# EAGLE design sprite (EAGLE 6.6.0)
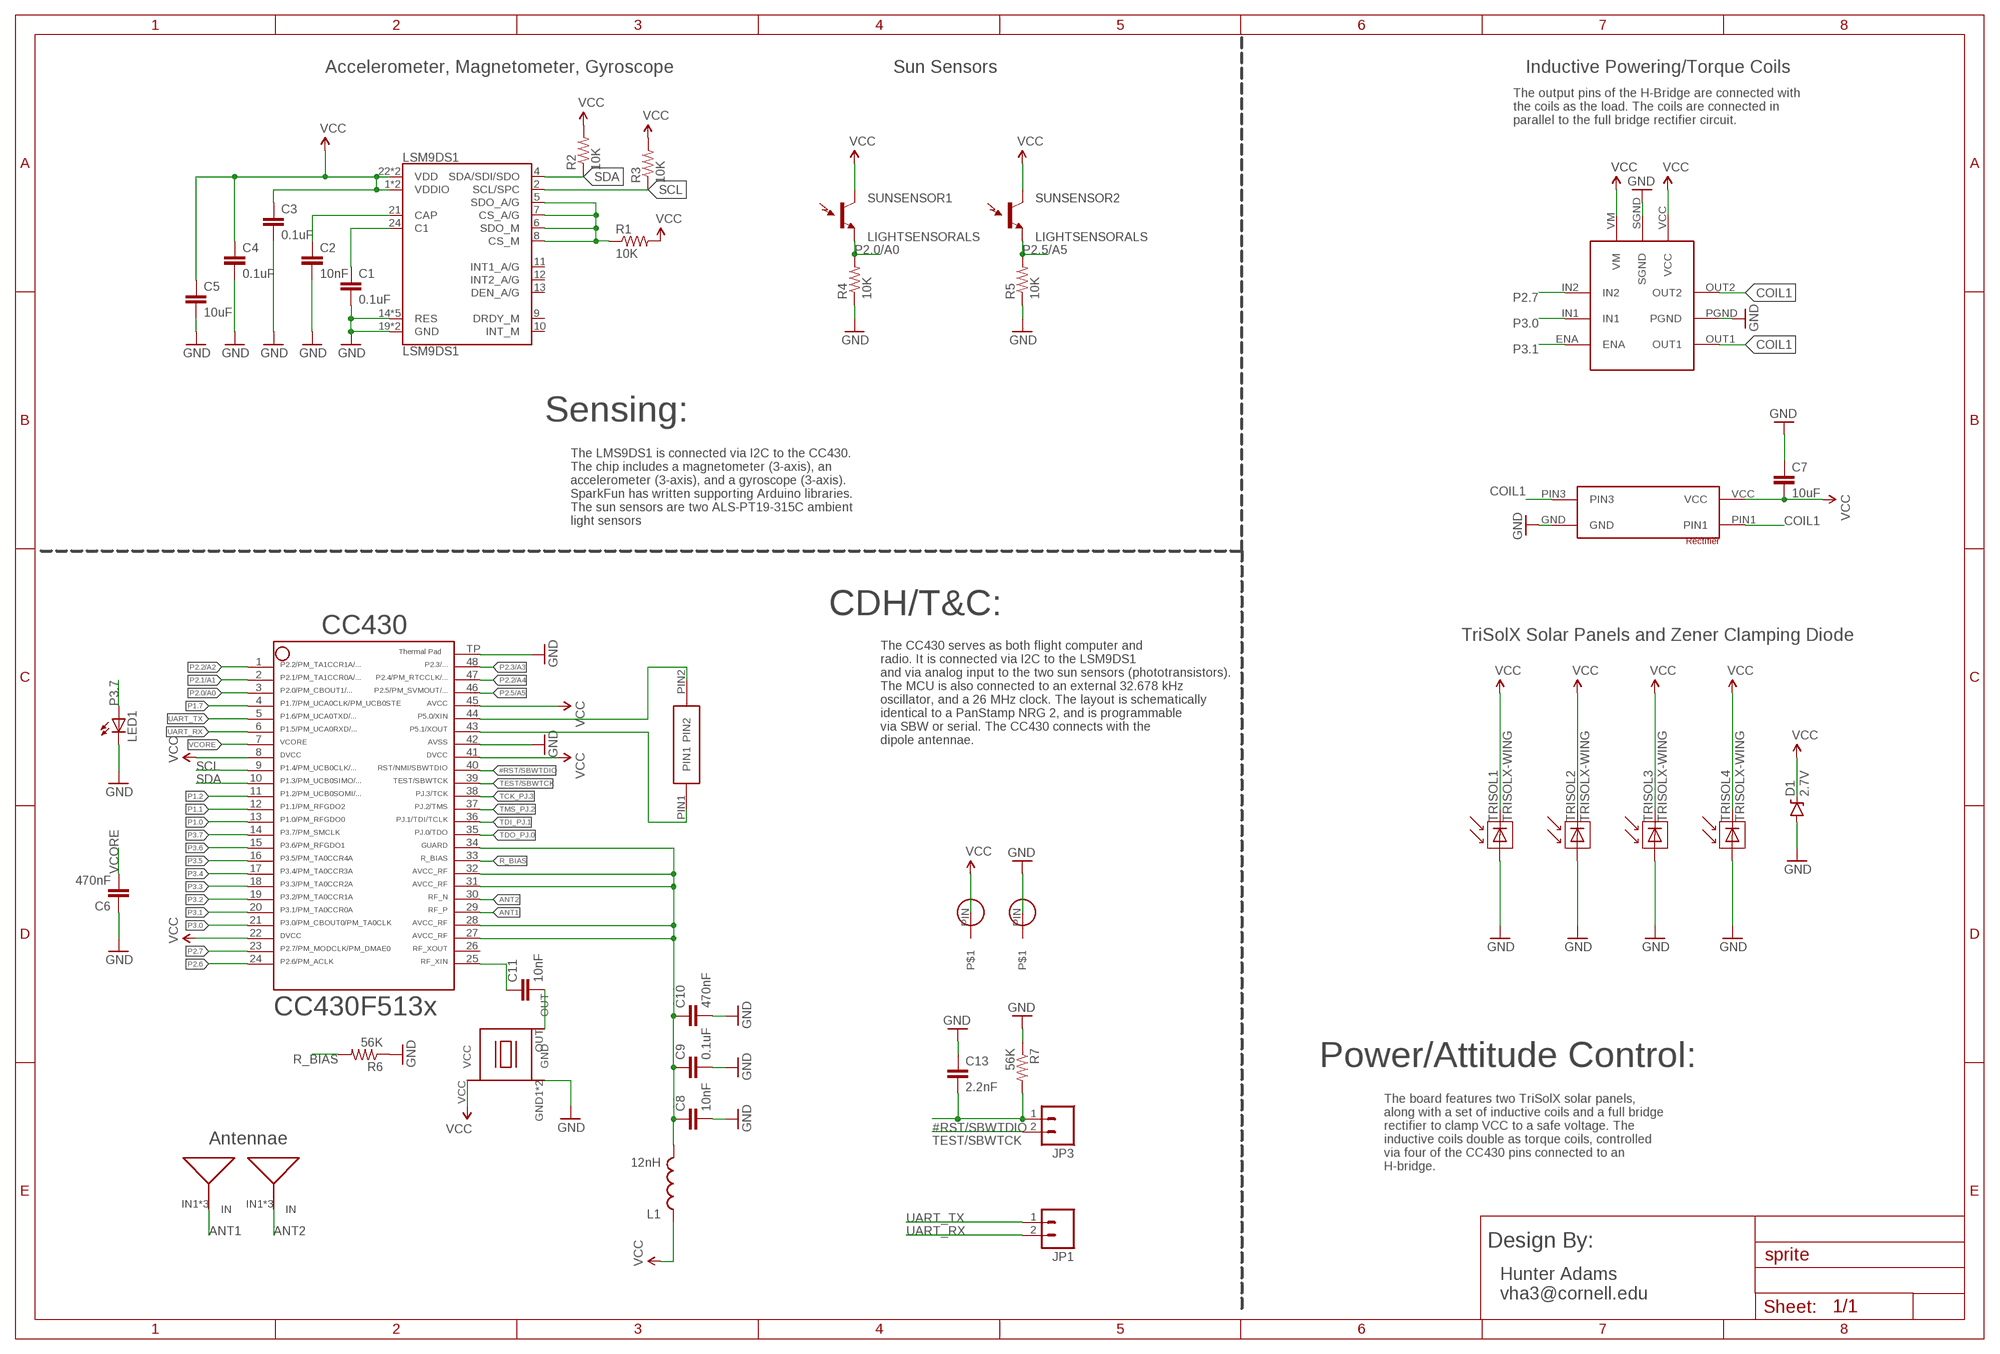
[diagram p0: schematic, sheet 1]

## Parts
32KHZ  SPRITECRYSTALSPRITECRYSTAL  [SPRITECRYSTAL]
ANTENNA1  ANTENNA  [ANTENNA]
ANTENNA2  ANTENNA  [ANTENNA]
C1  0.1uF  CAP0805  [0805]
C2  10nF  CAP0805  [0805]
C3  0.1uF  CAP0805  [0805]
C4  0.1uF  CAP0805  [0805]
C5  10uF  CAP0805  [0805]
C6  470nF  CAP0805  [0805]
C7  10uF  CAP0805  [0805]
C8  10nF  CAP0805  [0805]
C9  0.1uF  CAP0805  [0805]
C10  470nF  CAP0805  [0805]
C11  10nF  CAP0805  [0805]
C13  2.2nF  CAP0805  [0805]
CC430  CC430F513X---RGZ48  [RGZ48]
D1  2.7V  DIODE-ZENER3.3V  [SOD-323]
GNDPIN  SPRITE_PIN  [SPRITE_PIN]
H-BRIDGE  LV8417CS  [LV8417CS]
JP1  M02PTH  [1X02]
JP3  M02PTH  [1X02]
L1  12nH  INDUCTOR0402  [C0402]
LED1  LED0603  [LED-0603]
LSM9DS1  LSM9DS1  [LGA24-8X4]
R1  10K  RESISTOR0805-RES  [0805]
R2  10K  RESISTOR0805-RES  [0805]
R3  10K  RESISTOR0805-RES  [0805]
R4  10K  RESISTOR0805-RES  [0805]
R5  10K  RESISTOR0805-RES  [0805]
R6  56K  RESISTOR0805-RES  [0805]
R7  56K  RESISTOR0805-RES  [0805]
RECTIFIER  NSR1030QMUTAG  [NSR1030QMUTAG]
SUNSENSOR1  LIGHTSENSORALS  [ALS-PT19]
SUNSENSOR2  LIGHTSENSORALS  [ALS-PT19]
TRISOL1  TRISOLX-WING  [TRISOLX-T01]
TRISOL2  TRISOLX-WING  [TRISOLX-T01]
TRISOL3  TRISOLX-WING  [TRISOLX-T01]
TRISOL4  TRISOLX-WING  [TRISOLX-T01]
TXCO  TCXO_7Z  [TXC_7Z]
VCCPIN  SPRITE_PIN  [SPRITE_PIN]

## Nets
#RST/SBWTDIO: C13.2 CC430.40 JP3.1 R7.2
ANT1: ANTENNA1.IN1(IN) ANTENNA1.IN2(IN) ANTENNA1.IN3(IN) CC430.29
ANT2: ANTENNA2.IN1(IN) ANTENNA2.IN2(IN) ANTENNA2.IN3(IN) CC430.30
COIL1: H-BRIDGE.OUT1 H-BRIDGE.OUT2 RECTIFIER.PIN1 RECTIFIER.PIN3
GND: C1.2 C2.2 C3.2 C4.2 C5.2 C6.1 C7.1 C8.2 C9.2 C10.2 C13.1 CC430.42 CC430.TP D1.A GNDPIN.PIN H-BRIDGE.PGND H-BRIDGE.SGND LED1.C LSM9DS1.14(RES) LSM9DS1.15(RES) LSM9DS1.16(RES) LSM9DS1.17(RES) LSM9DS1.18(RES) LSM9DS1.19(GND) LSM9DS1.20(GND) R4.1 R5.1 R6.1 R7.1 RECTIFIER.GND TRISOL1.P$3(A) TRISOL2.P$3(A) TRISOL3.P$3(A) TRISOL4.P$3(A) TXCO.GND1(GND) TXCO.GND2(GND)
GUARD: C8.1 C9.1 C10.1 CC430.27 CC430.28 CC430.31 CC430.32 CC430.34 L1.2
N$1: C1.1 LSM9DS1.24(C1)
N$2: C2.1 LSM9DS1.21(CAP)
N$3: LSM9DS1.5(SDO_A/G) LSM9DS1.6(SDO_M) LSM9DS1.7(CS_A/G) LSM9DS1.8(CS_M) R1.1
N$4: C11.1 CC430.25
N$5: C11.2 TXCO.OUT
N$7: 32KHZ.PIN2 CC430.44
N$8: 32KHZ.PIN1 CC430.43
P1.0: CC430.13
P1.1: CC430.12
P1.2: CC430.11
P1.7: CC430.4
P2.0/A0: CC430.3 R4.2 SUNSENSOR1.E(E1)
P2.1/A1: CC430.2
P2.2/A2: CC430.1
P2.2/A4: CC430.47
P2.3/A3: CC430.48
P2.5/A5: CC430.46 R5.2 SUNSENSOR2.E(E1)
P2.6: CC430.24
P2.7: CC430.23 H-BRIDGE.IN2
P3.0: CC430.21 H-BRIDGE.IN1
P3.1: CC430.20 H-BRIDGE.ENA
P3.2: CC430.19
P3.3: CC430.18
P3.4: CC430.17
P3.5: CC430.16
P3.6: CC430.15
P3.7: CC430.14 LED1.A
R_BIAS: CC430.33 R6.2
SCL: CC430.9 LSM9DS1.2(SCL/SPC) R3.1
SDA: CC430.10 LSM9DS1.4(SDA/SDI/SDO) R2.1
TCK_PJ.3: CC430.38
TDI_PJ.1: CC430.36
TDO_PJ.0: CC430.35
TEST/SBWTCK: CC430.39 JP3.2
TMS_PJ.2: CC430.37
UART_RX: CC430.6 JP1.2
UART_TX: CC430.5 JP1.1
VCC: C3.1 C4.1 C5.1 C7.2 CC430.8 CC430.22 CC430.41 CC430.45 D1.C H-BRIDGE.VCC H-BRIDGE.VM L1.1 LSM9DS1.1(VDDIO) LSM9DS1.3(VDDIO) LSM9DS1.22(VDD) LSM9DS1.23(VDD) R1.2 R2.2 R3.2 RECTIFIER.VCC SUNSENSOR1.C(C1) SUNSENSOR2.C(C1) TRISOL1.P$2(C) TRISOL2.P$2(C) TRISOL3.P$2(C) TRISOL4.P$2(C) TXCO.VCC VCCPIN.PIN
VCORE: C6.2 CC430.7
Unconnected: CC430.26 LSM9DS1.9(DRDY_M) LSM9DS1.10(INT_M) LSM9DS1.11(INT1_A/G) LSM9DS1.12(INT2_A/G) LSM9DS1.13(DEN_A/G)

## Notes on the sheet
- Accelerometer, Magnetometer, Gyroscope | Sun Sensors | Inductive Powering/Torque Coils
- The output pins of the H-Bridge are connected with
  the coils as the load. The coils are connected in 
  parallel to the full bridge rectifier circuit.
- Sensing:
- The LMS9DS1 is connected via I2C to the CC430. 
  The chip includes a magnetometer (3-axis), an 
  accelerometer (3-axis), and a gyroscope (3-axis). 
  SparkFun has written supporting Arduino libraries. 
  The sun sensors are two ALS-PT19-315C ambient 
  light sensors
- CDH/T&C:
- TriSolX Solar Panels and Zener Clamping Diode
- The CC430 serves as both flight computer and
  radio. It is connected via I2C to the LSM9DS1 
  and via analog input to the two sun sensors (phototransistors). 
  The MCU is also connected to an external 32.678 kHz 
  oscillator, and a 26 MHz clock. The layout is schematically 
  identical to a PanStamp NRG 2, and is programmable 
  via SBW or serial. The CC430 connects with the 
  dipole antennae.
- Power/Attitude Control:
- Antennae
- The board features two TriSolX solar panels, 
  along with a set of inductive coils and a full bridge 
  rectifier to clamp VCC to a safe voltage. The 
  inductive coils double as torque coils, controlled 
  via four of the CC430 pins connected to an 
  H-bridge.
- Design By:
- Hunter Adams
  vha3@cornell.edu

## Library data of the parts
32KHZ = SpriteCrystal:SPRITECRYSTAL
ANTENNA1 ANTENNA2 = SpriteAntenna:ANTENNA
C1-C11 C13 = SparkFun:CAP: Capacitor
CC430 = TI_MSP430_v16:CC430F513X---RGZ48: ***CC430F513X***RGZ48 ** ** Rev 1.0 ** 06/2010 * http://focus.ti.com/docs/prod/folders/print/cc430f5137.html
D1 = SparkFun-DiscreteSemi:DIODE-ZENER: Zener Diode; PROD_ID: DIO-11284; VALUE: 3.3V
GNDPIN VCCPIN = SpritePin:SPRITE_PIN
H-BRIDGE = lv8417cs:LV8417CS
JP1 JP3 = SparkFun:M02: Header 2
L1 = SparkFun:INDUCTOR: Inductors
LED1 = SparkFun:LED: LEDs
LSM9DS1 = SparkFun-Sensors:LSM9DS1: LSM9DS1 3D accelerometer, gyroscope & magnetometer The LSM9DS1 is a system-in-package featuring a 3D digital linear acceleration sensor, a 3D digital angular rate sensor, and a 3D digital magnetic sensor. The LSM9DS1 has a linear acceleration full scale of ±2g/±4g/±8/±16 g, a magnetic field full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; PROD_ID: IC-12536
R1-R7 = SparkFun:RESISTOR: Resistor
RECTIFIER = NSR1030QMUTAG:NSR1030QMUTAG
SUNSENSOR1 SUNSENSOR2 = SparkFun-Sensors:LIGHTSENSOR: Ambient Light Sensor; PROD_ID: IC-11836
TRISOL1-TRISOL4 = TriSolX_QzQube:TRISOLX-WING
TXCO = SpriteTCXO:TCXO_7Z

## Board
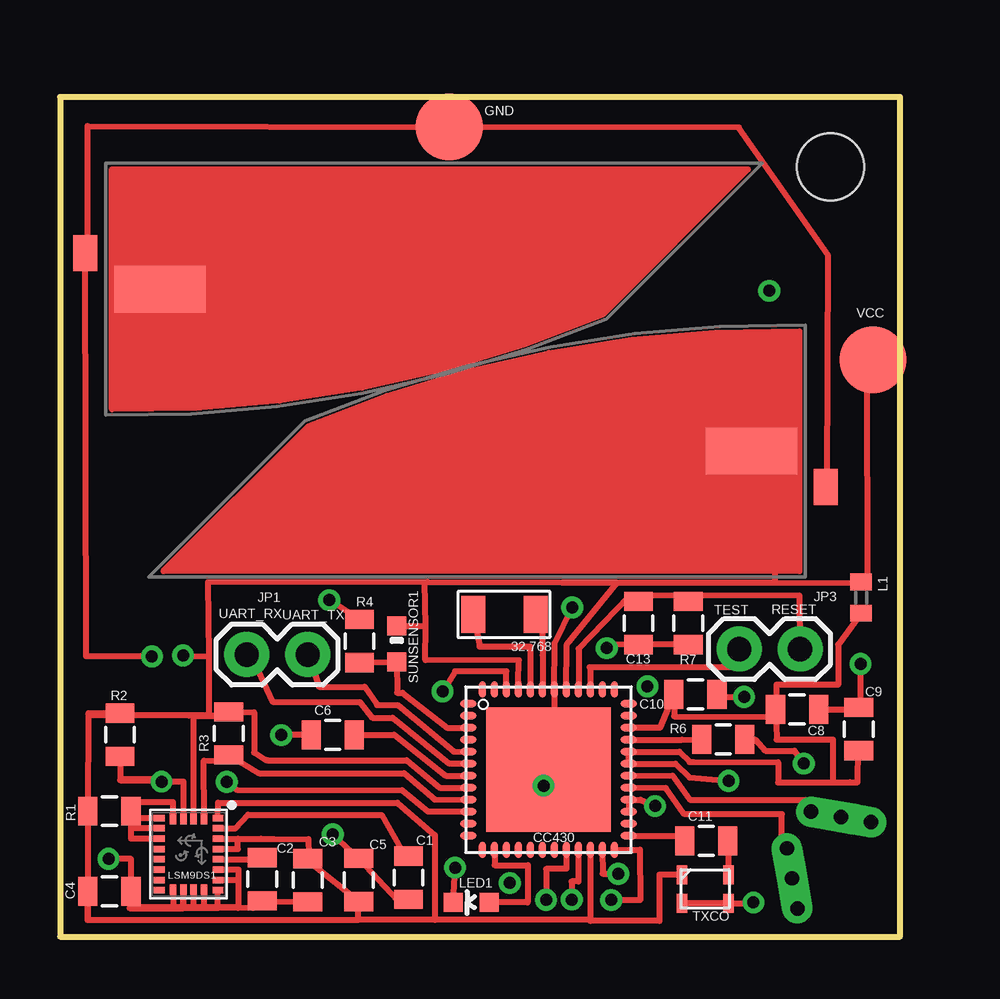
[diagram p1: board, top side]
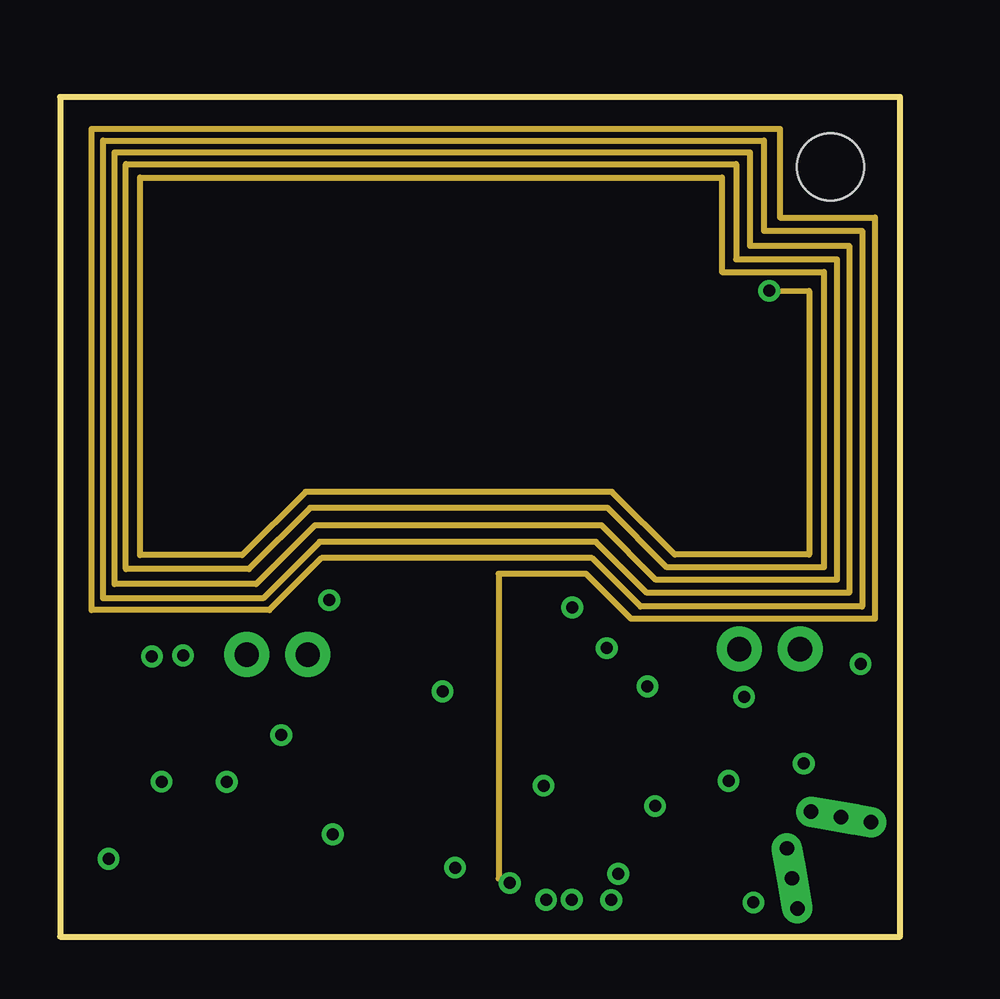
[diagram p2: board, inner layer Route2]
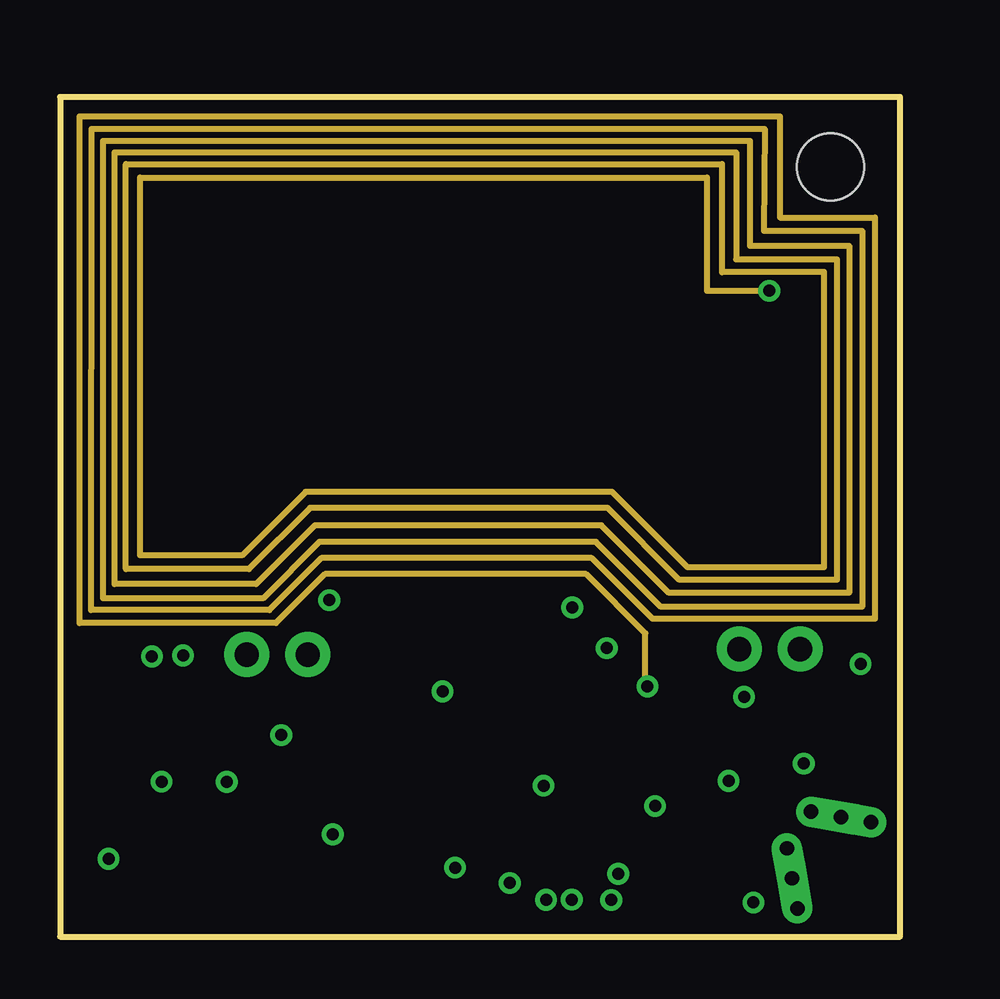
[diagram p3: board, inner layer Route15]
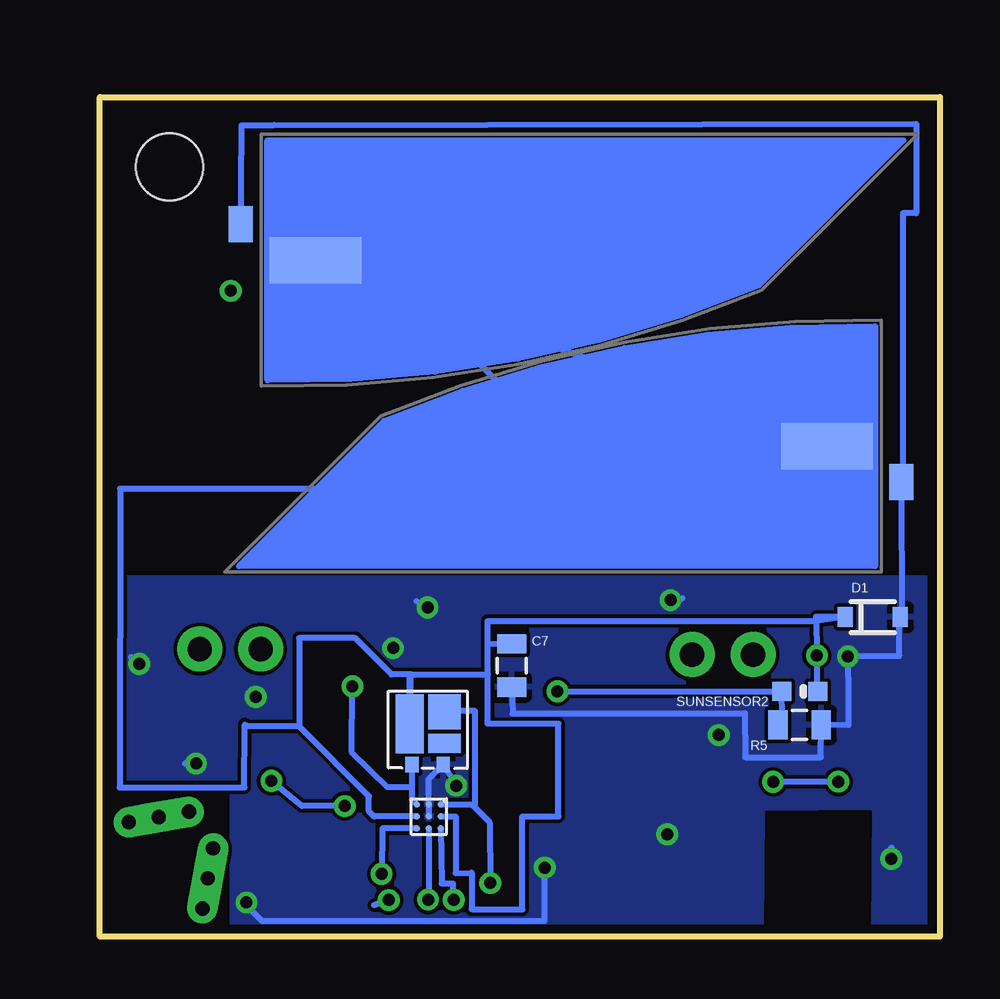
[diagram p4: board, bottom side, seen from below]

Size 35 x 35 mm. Coordinates in mm from the lower left corner, seen from the top.
Outline: 0,0 35,0 35,35 0,35 0,0
Copper layers (1*2*15*16): Top 0.035559375mm / dielectric 1.501140625mm / Route2 0.035559375mm / dielectric 0.149859375mm / Route15 0.035559375mm / dielectric 0.200659375mm / Bottom 0.035559375mm
Design rules "typical_4pcb *": minimum track width 10mil, minimum drill 15mil, track to track 6mil, track to pad 6mil, pad to pad 6mil, via to via 6mil, smd to smd 6mil, copper to edge 15mil, drill to drill 8mil, minimum pad ring 10mil, minimum via ring 8mil, stop-mask expansion 4mil, vias tented up to drill 0mil, thermal gap 10mil
Holes 2.8 mm at 32.1,32.1

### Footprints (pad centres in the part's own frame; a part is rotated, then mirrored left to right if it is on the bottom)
SPRITECRYSTAL = smd 1 x 1.55: PIN1 -1.3,0; PIN2 1.3,0
ANTENNA = drill 0.6 pad 1.27 square: IN1 0,0 | drill 0.6 pad 1.27 offset: IN2 1.27,0; IN3 -1.27,0
0805 = smd 0.8 x 1.2: 1 -0.9,0; 2 0.9,0
RGZ48 = smd 0.7 x 0.3: 1 -3.35,2.75; 2 -3.35,2.25; 3 -3.35,1.75; 4 -3.35,1.25; 5 -3.35,0.75; 6 -3.35,0.25; 7 -3.35,-0.25; 8 -3.35,-0.75; 9 -3.35,-1.25; 10 -3.35,-1.75; 11 -3.35,-2.25; 12 -3.35,-2.75; 25 3.35,-2.75; 26 3.35,-2.25; 27 3.35,-1.75; 28 3.35,-1.25; 29 3.35,-0.75; 30 3.35,-0.25; 31 3.35,0.25; 32 3.35,0.75; 33 3.35,1.25; 34 3.35,1.75; 35 3.35,2.25; 36 3.35,2.75 | smd 0.3 x 0.7: 13 -2.75,-3.35; 14 -2.25,-3.35; 15 -1.75,-3.35; 16 -1.25,-3.35; 17 -0.75,-3.35; 18 -0.25,-3.35; 19 0.25,-3.35; 20 0.75,-3.35; 21 1.25,-3.35; 22 1.75,-3.35; 23 2.25,-3.35; 24 2.75,-3.35; 37 2.75,3.35; 38 2.25,3.35; 39 1.75,3.35; 40 1.25,3.35; 41 0.75,3.35; 42 0.25,3.35; 43 -0.25,3.35; 44 -0.75,3.35; 45 -1.25,3.35; 46 -1.75,3.35; 47 -2.25,3.35; 48 -2.75,3.35 | smd 5.2 x 5.2: TP 0,0
SOD-323 = smd 0.63 x 0.83: A 1.15,0; C -1.15,0
SPRITE_PIN = smd 2.794 x 2.794: PIN 0,0
LV8417CS = smd 0.27 x 0.27: ENA 0.5,-0.5; IN1 0,-0.5; IN2 -0.5,-0.5; OUT1 0.5,0.5; OUT2 -0.5,0.5; PGND 0,0.5; SGND 0,0; VCC 0.5,0; VM -0.5,0
1X02 = drill 1.016 pad 1.88: 1 0,0; 2 2.54,0
C0402 = smd 0.7 x 0.9: 1 -0.65,0; 2 0.65,0
LED-0603 = smd 0.8 x 0.8: A 0,-0.75; C 0,0.75
LGA24-8X4 = smd 0.27 x 0.45: 1 -1.505,1.225; 6 -1.505,-1.225; 7 -1.075,-1.225; 8 -0.645,-1.225; 9 -0.215,-1.225; 10 0.215,-1.225; 11 0.645,-1.225; 12 1.075,-1.225; 13 1.505,-1.225; 18 1.505,1.225; 19 1.075,1.225; 20 0.645,1.225; 21 0.215,1.225; 22 -0.215,1.225; 23 -0.645,1.225; 24 -1.075,1.225 | smd 0.45 x 0.27: 2 -1.475,0.645; 3 -1.475,0.215; 4 -1.475,-0.215; 5 -1.475,-0.645; 14 1.475,-0.645; 15 1.475,-0.215; 16 1.475,0.215; 17 1.475,0.645
NSR1030QMUTAG = smd 0.55 x 0.633: GND -0.65,1.335; PIN3 0.65,1.335 | smd 1.35 x 0.8: P$2 -0.706,0.453 | smd 1.35 x 1.45: PIN1 -0.7,-0.865 | smd 1.15 x 2.45: VCC 0.738,-0.365
ALS-PT19 = smd 0.8 x 0.8: C -0.75,0; E 0.75,0
TRISOLX-T01 = smd 3.81 x 1.93: P$2 -2,5 | smd 1 x 1.5: P$3 1.1,3.5
TXC_7Z = smd 0.44 x 0.79: GND1 -0.97,-0.595; GND2 0.97,-0.595; OUT 0.97,0.595; VCC -0.97,0.595

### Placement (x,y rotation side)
32KHZ  18.52,13.44 180 top
ANTENNA1  30.51,2.44 100 top
ANTENNA2  32.55,5 170 top
C1  14.52,2.47 270 top
C2  8.43,2.4 270 top
C3  10.32,2.36 270 top
C4  2.06,1.9 0 top
C5  12.45,2.37 90 top
C6  11.36,8.41 0 top
C7  17.84,11.31 90 bottom
C8  30.71,9.48 0 top
C9  33.28,8.66 90 top
C10  26.48,10.11 0 top
C11  26.93,4 0 top
C13  24.11,13.08 90 top
CC430  20.35,6.97 0 top
D1  2.8,13.33 0 bottom
GNDPIN  16.22,33.76 0 top
H-BRIDGE  21.29,5.02 0 bottom
JP1  10.32,11.77 180 top
JP3  30.84,11.99 180 top
L1  33.38,14.14 270 top
LED1  17.13,1.44 90 top
LSM9DS1  5.36,3.45 270 top
R1  2.06,5.24 180 top
R2  2.5,8.42 90 top
R3  7.03,8.48 90 top
R4  12.48,12.32 270 top
R5  5.85,8.83 180 bottom
R6  27.63,8.22 180 top
R7  26.18,13.08 90 top
RECTIFIER  21.35,8.51 180 bottom
SUNSENSOR1  14.04,12.2 270 top
SUNSENSOR2  5.84,10.23 180 bottom
TRISOL1  2.16,31.99 180 top
TRISOL2  30.81,15.24 0 top
TRISOL3  2.7,15.45 0 bottom
TRISOL4  28.03,33.2 180 bottom
TXCO  26.88,2 0 top
VCCPIN  33.87,24.05 0 top

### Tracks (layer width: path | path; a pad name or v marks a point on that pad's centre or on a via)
#RST/SBWTDIO
  Top 0.254: R7.2 25.97,13.98 25.97,14.21 24.61,14.22 C13.2 23.7,14.18 | 23.7,14.18 21.61,12.01 21.61,10.32 CC430.40 | JP3.1 30.82,14.22 24.43,14.21 24.28,14.06 23.7,14.18
ANT1
  Top 0.254: ANTENNA1.IN3 ANTENNA1.IN1 ANTENNA1.IN2 30.08,3.64 30.08,5.11 26.02,5.11 25.24,6.2 23.72,6.2 CC430.29
ANT2
  Top 0.254: ANTENNA2.IN3 ANTENNA2.IN1 ANTENNA2.IN2 31.29,5.7 26.25,5.71 25.52,6.73 CC430.30
COIL1  (via drill 0.5)
  Route2 0.254: v18.74,2.24 18.28,2.43 18.28,15.13 21.92,15.13 23.79,13.26 33.95,13.26 33.95,29.99 30,29.99 30,33.68 1.32,33.68 1.32,13.62 8.72,13.62 10.89,15.79 22.17,15.79 24.2,13.76 33.42,13.76 33.42,29.43 29.33,29.43 29.33,33.19 1.8,33.19 1.8,14.11 8.46,14.11 10.81,16.46 22.33,16.46 24.46,14.34 32.88,14.34 32.88,28.81 28.74,28.81 28.74,32.7 2.27,32.7 2.27,14.7 8.17,14.7 10.62,17.15 22.56,17.15 24.83,14.88 32.37,14.88 32.37,28.24 28.17,28.24 28.17,32.21 2.75,32.21 2.75,15.33 7.87,15.33 10.42,17.88 22.82,17.88 25.29,15.4 31.83,15.4 31.83,27.71 27.57,27.71 27.57,31.65 3.34,31.65 3.34,15.91 7.59,15.91 10.23,18.55 23,18.55 25.62,15.93 | v29.55,26.93 31.21,26.92 31.21,15.93 25.62,15.93 | 25.62,15.93
  Route15 0.254: v24.48,10.44 24.39,10.51 | 24.39,10.51 24.23,10.63 | 24.39,10.51 24.39,12.65 21.92,15.12 | 21.92,15.12 | 21.92,15.12 11.04,15.12 9,13.08 0.82,13.08 0.82,34.21 29.99,34.21 29.99,29.99 33.96,29.99 33.96,13.26 24.69,13.26 22.17,15.78 10.88,15.78 8.72,13.62 1.29,13.62 1.32,33.68 29.36,33.68 29.33,29.43 33.42,29.43 33.42,13.76 25.03,13.76 22.33,16.46 10.81,16.46 8.46,14.11 1.8,14.11 1.8,33.19 28.74,33.19 28.74,28.8 32.88,28.8 32.88,14.34 25.37,14.34 22.56,17.15 10.62,17.15 8.17,14.7 2.27,14.7 2.27,32.7 28.17,32.7 28.17,28.24 32.37,28.24 32.37,14.88 25.81,14.88 22.82,17.88 10.42,17.88 7.87,15.33 2.75,15.33 2.75,32.21 27.58,32.21 27.58,27.72 | 27.58,27.72 27.58,27.69 | 27.58,27.72 31.83,27.72 31.83,15.4 26.15,15.4 23.01,18.55 10.23,18.55 7.59,15.9 3.34,15.9 3.34,31.65 26.95,31.65 26.95,26.93 v29.55,26.93
  Bottom 0.254: H-BRIDGE.OUT1 19.5,5.51 | 19.5,5.51 19.36,5.51 19.36,9.41 20.65,9.41 RECTIFIER.PIN1 | 19.5,5.51 18.77,4.77 v18.74,2.24 | 22,6.24 22,5.72 H-BRIDGE.OUT2 | 22,6.24 23.02,6.24 24.5,7.68 v24.48,10.44 | RECTIFIER.PIN3 22,6.24
GND  (via drill 0.5)
  Top 0.254: 6.55,1.97 LSM9DS1.18 6.58,1.2 | 7.42,1.19 8.05,1.2 8.06,1.5 C2.2 8.21,1.48 C3.2 | 7.42,1.19 6.58,1.2 | C1.2 14.08,1.52 C5.2 v11.36,4.27 | C4.2 2.9,1.2 4.69,1.2 | 4.69,1.2 5.14,1.2 LSM9DS1.15 5.13,1.2 5.56,1.2 | C9.2 33.65,9.48 C8.2 33.36,9.48 v33.36,11.37 | R7.1 C13.1 22.89,12.18 v22.79,12.04 | 7.43,2.37 7.43,2.8 LSM9DS1.20 7.42,2.8 7.42,1.22 2.96,1.22 2.96,3.25 v2.02,3.25 | 7.43,2.37 7.42,1.19 | LSM9DS1.19 7.43,2.37 | LSM9DS1.14 4.71,1.22 4.69,1.2 | 5.56,1.2 5.99,1.2 | 5.99,1.2 6.58,1.2 | LSM9DS1.16 5.56,1.2 | LSM9DS1.17 5.99,1.2 | TRISOL2.P$3 31.97,18.94 32.01,28.42 28.29,33.73 16.32,33.74 GNDPIN.PIN 1.15,33.8 1.15,28.65 TRISOL1.P$3 1.09,11.69 v3.83,11.69 | v21.35,13.73 20.61,12.23 CC430.42 20.6,9.3 20.59,9.3 CC430.TP 20.35,6.43 20.09,6.17 v20.15,6.3 | LED1.C v16.46,2.88 | C6.1 v9.21,8.41 | R4.1 v11.22,14.04 | C10.2 27.55,10.01 v28.5,10 | R6.1 28.96,8.22 29.39,7.75 30.6,7.75 v30.99,7.22 | 28.93,1.45 v28.89,1.43 28.96,1.4 TXCO.GND2 TXCO.GND1
  Bottom 0.254: C7.1 17.81,9.31 8.13,9.32 8.12,7.49 4.96,7.48 R5.1 3.82,8.81 3.82,10 v3.83,11.69 1.7,11.69 1.71,11.79 1.71,13.41 1.79,13.42 D1.A 1.59,13.24 TRISOL3.P$3 1.36,18.9 1.54,18.67 1.54,30.16 0.99,30.16 0.99,33.89 27.75,33.83 29.1,33.83 29.11,31.3 29.12,29.47 29.22,29.61 TRISOL4.P$3 | H-BRIDGE.SGND H-BRIDGE.PGND 21.29,6.59 RECTIFIER.GND v20.15,6.3 | 16.41,2.92 v16.46,2.88 16.47,0.66 16.62,0.66 28.25,0.66 29.04,1.44 v28.89,1.43 | v11.36,4.27 11.27,4.42 | v9.21,8.41 8.99,8.64 | v11.22,14.04 10.73,14.11 | v2.02,3.25 2.02,3.72 | v21.35,13.73 21.8,13.98 | v22.79,12.04 22.81,11.89 | v28.5,10 28.44,9.85 | v30.99,7.22 31.46,7.22 | v33.36,11.37 33.71,11.66
  pour Bottom: 0.21,14.95 34.8,14.95 34.8,6.09 29.49,6.09 29.49,0.25 7.44,0.21 7.41,5.38 2.72,5.42 2.76,0.12 -0.17,0.14 -0.17,14.97
GUARD  (via drill 0.5)
  Top 0.254: CC430.27 CC430.28 24.2,5.72 v24.8,5.45 | CC430.34 24.99,8.72 C10.1 25.59,9.19 29.86,9.17 | 29.86,9.17 29.86,9.08 C8.1 29.86,8.22 32.2,8.22 32.2,6.45 32.92,6.44 | L1.2 32.42,12.17 32.42,10.51 29.85,10.51 29.84,9.24 29.89,9.03 29.86,9.17 | 32.92,6.44 33.23,6.44 33.24,6.95 C9.1 | 32.92,6.44 29.92,6.44 29.92,7.28 26.4,7.29 26.24,7.29 25.81,7.72 CC430.32 CC430.31 25.64,7.22 26.22,6.64 v27.86,6.5
  Bottom 0.254: 27.78,6.66 v27.86,6.5 26.59,5.45 v24.8,5.45
N$1
  Top 0.254: LSM9DS1.24 6.56,4.53 7.3,4.52 7.83,5.09 13.4,5.08 14.22,3.65 14.36,3.37 C1.1
N$2
  Top 0.254: LSM9DS1.21 8,3.22 C2.1
N$3
  Top 0.254: 4.1,4.92 LSM9DS1.6 2.9,4.95 R1.1 | LSM9DS1.8 2.96,4.09 2.96,4.52 | 2.96,4.52 R1.1 | LSM9DS1.7 2.96,4.52 | LSM9DS1.5 4.71,5.61 3.33,5.61 arc90 R1.1
N$4
  Top 0.254: CC430.25 26.03,4.22 C11.1
N$5
  Top 0.254: C11.2 27.85,4 TXCO.OUT
N$7
  Top 0.254: 32KHZ.PIN2 17.49,12.09 19.6,12.09 CC430.44 | CC430.44
N$8
  Top 0.254: 32KHZ.PIN1 19.95,13.28 19.93,13.23 20.07,13.37 20.11,11.73 CC430.43
P2.0/A0
  Top 0.254: CC430.3 16.13,8.71 14.27,10.17 14.04,10.17 SUNSENSOR1.E 13.97,11.43 R4.2
P2.5/A5  (via drill 0.5)
  Top 0.254: CC430.46 18.6,11.06 16.46,11.06 v15.94,10.23
  Bottom 0.254: R5.2 6.58,9.19 SUNSENSOR2.E 6.55,10.23 v15.94,10.23
P2.6  (via drill 0.5)
  Top 0.254: CC430.24 24.17,3.63 24.18,1.53 23.31,1.52 v22.97,1.53
  Bottom 0.254: v22.97,1.53 23.57,1.32
P2.7  (via drill 0.5)
  Top 0.254: CC430.23 22.61,2.63 v23.26,2.63
  Bottom 0.254: 23.4,2.47 v23.26,2.63 23.23,4.51 H-BRIDGE.IN2
P3.0  (via drill 0.5)
  Top 0.254: CC430.21 21.6,2.31 21.32,2.3 v21.33,1.55
  Bottom 0.254: 21.43,1.55 v21.33,1.55 21.29,1.75 H-BRIDGE.IN1
P3.1  (via drill 0.5)
  Top 0.254: CC430.20 21.1,2.84 20.25,2.83 v20.25,1.54
  Bottom 0.254: H-BRIDGE.ENA 20.76,2.22 20.29,2.22 20.29,1.52 20.16,1.54 v20.25,1.54
P3.7
  Top 0.254: CC430.14 18.11,3.62 18.11,2.98 19.49,2.98 19.49,1.45 19.48,1.44 LED1.A
R_BIAS
  Top 0.254: CC430.33 25.91,8.22 R6.2
SCL
  Top 0.254: LSM9DS1.2 6,7.35 6.87,7.33 7.27,7.45 R3.1 8.3,6.82 14.34,6.82 15.61,5.72 CC430.9
SDA  (via drill 0.5)
  Top 0.254: LSM9DS1.4 5.14,6.48 v4.23,6.47 4.18,6.53 2.51,6.53 R2.1 2.51,6.58 4.19,6.58 v4.23,6.47 | v6.95,6.46 7.36,6.13 14.25,6.11 15.32,5.23 CC430.10
  Bottom 0.254: v4.23,6.47 v6.95,6.46
TEST/SBWTCK
  Top 0.254: JP3.2 28.28,11.23 22.07,11.23 22.1,11.18 CC430.39
UART_RX
  Top 0.254: JP1.2 7.89,11.91 8.86,9.79 12.5,9.79 13.02,9.13 13.86,9.13 16.19,7.23 CC430.6
UART_TX
  Top 0.254: JP1.1 10.8,10.42 12.68,10.42 12.69,10.41 13.21,9.66 14.07,9.66 16.4,7.72 16.99,7.71 CC430.5
VCC  (via drill 0.5)
  Top 0.254: 15.3,14.8 20.91,14.76 | 20.91,14.76 29.79,14.76 | 29.79,14.76 33.66,14.76 | 33.66,14.76 33.63,23.63 VCCPIN.PIN | 33.66,14.76 33.3,14.84 L1.1 | CC430.8 16.98,6.2 15.82,6.21 14.44,7.36 8.64,7.36 8.57,7.38 8.09,7.68 8.09,9.36 R3.2 7.24,9.3 7.25,9.21 5.57,9.23 LSM9DS1.3 5.58,9.22 7.12,9.21 5.38,9.22 2.95,9.22 2.53,9.31 R2.2 1.18,9.31 | 1.15,0.71 R1.2 1.18,9.31 | 1.15,0.71 C4.1 | 15.3,14.8 6.16,14.78 6.2,11.68 | 6.2,11.68 6.2,9.22 1.2,9.22 1.18,9.31 | CC430.41 21.12,12.2 23.23,14.77 20.91,14.76 | SUNSENSOR1.C 15.23,12.95 | 15.23,12.95 15.2,14.77 15.3,14.8 | CC430.45 19.1,10.61 19.12,11.52 15.23,11.54 15.23,12.95 | 1.15,0.71 12.42,0.7 | 12.42,0.7 C5.1 10.5,3.01 C3.1 10.3,3.24 10.36,3.43 10.35,4.07 8.91,4.08 8.37,4.09 7.41,4.08 | LSM9DS1.23 7.41,4.08 | CC430.22 22.1,0.7 | 22.1,0.7 15.62,0.7 | 15.62,0.7 12.42,0.7 | LSM9DS1.1 6.59,5.59 14.05,5.59 15.62,4.24 15.62,0.7 | v5.12,11.73 5.12,11.7 5.13,11.71 6.2,11.68 | 29.79,22.51 29.79,14.76 | LSM9DS1.22 7.41,3.66 7.41,4.08 | TXCO.VCC 24.97,2.59 24.97,0.66 22.1,0.66 22.1,0.7
  Top 0.406: TRISOL2.P$2 TRISOL1.P$2 21.21,22.51 29.79,22.51
  Bottom 0.254: SUNSENSOR2.C v5.12,11.73 5.16,13.34 | 4.14,13.32 5.12,13.16 | 5.12,13.16 5.16,13.34 | D1.C 4.25,13.32 5.16,13.34 | 5.12,13.16 13.68,13.16 18.85,13.16 18.84,12.17 18.84,12.19 | C7.2 18.84,12.19 | 23.56,5.01 H-BRIDGE.VM 23.59,5.01 23.79,5.22 23.79,5.85 26.7,8.76 | 22.1,8.87 RECTIFIER.VCC | H-BRIDGE.VCC 20.18,5.01 20.18,2.65 19.51,2.67 19.51,1.15 18.84,1.14 17.4,1.14 17.4,5.01 15.89,5.01 15.89,8.88 18.84,8.88 18.84,9.42 18.84,10.94 | 18.84,10.94 18.84,12.19 | TRISOL3.P$2 TRISOL4.P$2 22.46,27.17 13.96,18.67 34.16,18.67 34.18,6.22 28.98,6.22 28.95,8.76 | 22.05,8.88 22.05,10.94 18.84,10.94 | 28.95,8.76 28.95,8.85 | 26.7,8.76 28.95,8.76 | RECTIFIER.VCC 22.09,10.93 22.85,10.93 24.36,12.45 26.7,12.45 26.7,8.76 | RECTIFIER.VCC 22.05,8.88 | 22.05,8.88 22.05,8.86
VCORE
  Top 0.254: C6.2 13.92,8.42 16.08,6.71 17,6.71 CC430.7

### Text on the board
tPlace: GND | VCC | UART_RX | UART_TX | TEST | RESET

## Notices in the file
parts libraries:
SparkFun-Sensors: Licensing: Creative Commons ShareAlike 4.0 International - https://creativecommons.org/licenses/by-sa/4.0
SparkFun: Licensing: CC v3.0 Share-Alike You are welcome to use this library for commercial purposes.
